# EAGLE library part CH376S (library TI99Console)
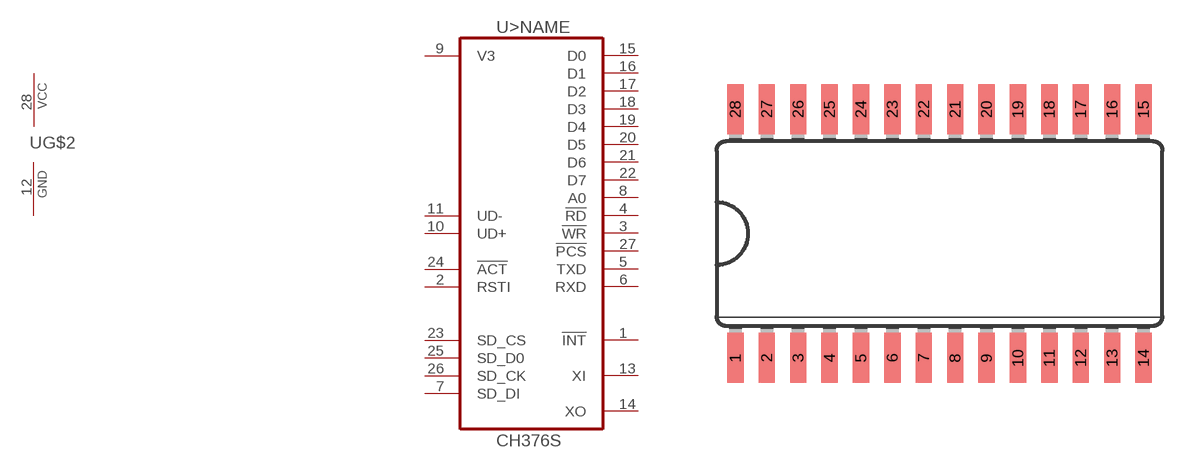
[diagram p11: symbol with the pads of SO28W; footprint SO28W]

Designator prefix -; gates >NAME=CH376S G$2=74XX-US_PWRN

## CH376SPIO  [SO28W]
1  >NAME:!INT  out
2  >NAME:RSTI  in
3  >NAME:!WR  in
4  >NAME:!RD  in
5  >NAME:TXD  pas
6  >NAME:RXD  pas
7  >NAME:SD_DI  in
8  >NAME:A0  in
9  >NAME:V3  hiz
10  >NAME:UD+  hiz
11  >NAME:UD-  hiz
12  G$2:GND  pwr
13  >NAME:XI  pas
14  >NAME:XO  pas
15  >NAME:D0
16  >NAME:D1
17  >NAME:D2
18  >NAME:D3
19  >NAME:D4
20  >NAME:D5
21  >NAME:D6
22  >NAME:D7
23  >NAME:SD_CS  out
24  >NAME:!ACT  in
25  >NAME:SD_D0  out
26  >NAME:SD_CK  out
27  >NAME:!PCS  in
28  G$2:VCC  pwr

## Footprint SO28W (pad centres in mm)
smd 0.66 x 2.032: 1 -6.985,-1.219; 2 -5.715,-1.219; 3 -4.445,-1.219; 4 -3.175,-1.219; 5 -1.905,-1.219; 6 -0.635,-1.219; 7 0.635,-1.219; 8 1.905,-1.219; 9 3.175,-1.219; 10 4.445,-1.219; 11 5.715,-1.219; 12 6.985,-1.219; 13 8.255,-1.219; 14 9.525,-1.219; 15 9.525,8.839; 16 8.255,8.839; 17 6.985,8.839; 18 5.715,8.839; 19 4.445,8.839; 20 3.175,8.839; 21 1.905,8.839; 22 0.635,8.839; 23 -0.635,8.839; 24 -1.905,8.839; 25 -3.175,8.839; 26 -4.445,8.839; 27 -5.715,8.839; 28 -6.985,8.839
